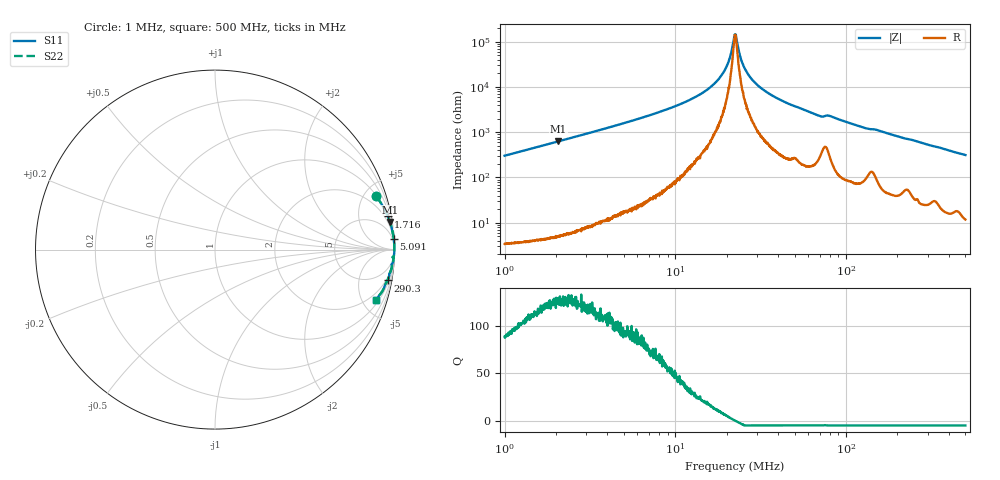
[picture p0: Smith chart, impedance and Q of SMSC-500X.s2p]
!s-Parameter Generated by FASTRON Sdn. Bhd.
!FASTRON P/N : SMSC-500X
!Keysight Technologies,E4991B,MY54100416,A.01.15
!Date: Thu Mar 19 12:55:35 2026
!Version  : Rev00 Thu Mar 19 12:55:35 2026
!Data & Calibration Information:
!PortZ  Port1:50+j0  Port2:50+j0
!When reading, reference impedance value at option line is always used.
! Remarks : This data is being provided solely for informational purposes.
!Freq	S11	S21	S12	S22
# Hz S dB R 50
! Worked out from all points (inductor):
!   1601 points, 1 MHz to 500 MHz, reference 50 ohm
!   read as one part in series: L = 48 uH near 1.032 MHz
!   highest Q = 128 at 2.067 MHz (marker M1), where L = 48.5 uH
!   self-resonance near 22.36 MHz
!   S11 on the Smith chart (normalised r, x): 1 MHz: 1.07, +6.05; 1.716 MHz: 1, +10; 5.091 MHz: 1, +32; 290.3 MHz: 1, -11; 500 MHz: 1.24, -6.27
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1000000  -0.48 18.2  -10.10 -71.1  -10.10 -71.1  -0.48 18.2
1715825  -0.17 10.8  -14.51 -78.7  -14.51 -78.7  -0.17 10.8
2067484  -0.12 9.0  -16.10 -80.5  -16.10 -80.5  -0.12 9.0
2820919  -0.07 6.6  -18.81 -82.9  -18.81 -82.9  -0.07 6.6
5090879  -0.02 3.5  -24.21 -85.9  -24.21 -85.9  -0.02 3.5
7957584  -0.01 2.1  -28.80 -87.1  -28.80 -87.1  -0.01 2.1
1.263331e7  -0.01 1.0  -34.93 -87.1  -34.93 -87.1  -0.01 1.0
1.684009e7  -0.01 0.5  -41.30 -85.3  -41.30 -85.3  -0.01 0.5
1.982405e7  -0.01 0.2  -48.52 -79.3  -48.52 -79.3  -0.01 0.2
2.06894e7  -0.01 0.1  -51.97 -74.8  -51.97 -74.8  -0.01 0.1
2.193061e7  -0.01 0.0  -60.39 -41.4  -60.39 -41.4  -0.01 0.0
2.236068e7  -0.01 0.0  -62.73 -7.8  -62.73 -7.8  -0.01 0.0
2.288791e7  -0.01 -0.0  -60.76 39.2  -60.76 39.2  -0.01 -0.0
2.416697e7  -0.01 -0.1  -52.75 71.4  -52.75 71.4  -0.01 -0.1
2.541858e7  -0.01 -0.2  -48.43 78.3  -48.43 78.3  -0.01 -0.2
2.980659e7  -0.01 -0.5  -41.32 83.8  -41.32 83.8  -0.01 -0.5
4.004179e7  -0.01 -1.0  -34.80 85.4  -34.80 85.4  -0.01 -1.0
6.307767e7  -0.03 -2.1  -28.56 84.1  -28.56 84.1  -0.03 -2.1
7.994179e7  -0.06 -2.5  -27.30 80.1  -27.30 80.1  -0.06 -2.5
1.77937e8  -0.09 -6.1  -19.43 81.1  -19.43 81.1  -0.09 -6.1
2.902753e8  -0.21 -10.1  -15.08 77.3  -15.08 77.3  -0.21 -10.1
5e8  -0.51 -17.5  -10.45 70.4  -10.45 70.4  -0.51 -17.5
